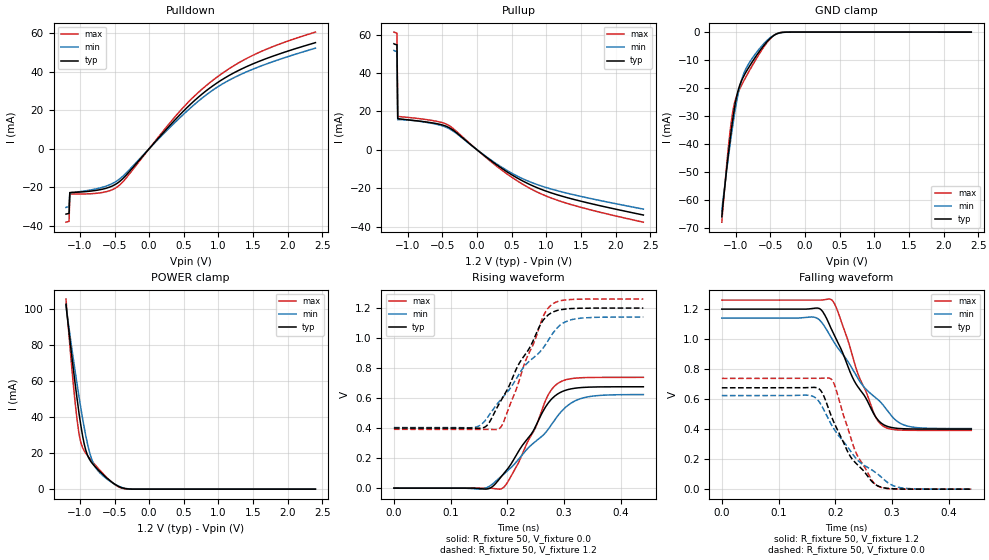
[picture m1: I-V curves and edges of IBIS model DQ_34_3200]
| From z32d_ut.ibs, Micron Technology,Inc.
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| MODEL DQ_34_3200 (34 Ohm Data I/O with no ODT, 1600-3200Mbps)
[Model]   DQ_34_3200
Model_type   I/O
Vinl = 905.000mV
Vinh = 1015.000mV
Vmeas = 960.000mV
Vref = 1200.000mV
Cref = 0.0pF
Rref = 50.000Ohm
|   typ   min   max
|C_comp   0.636pF   0.586pF   0.686pF
C_comp_pullup   0.318pF   0.293pF   0.343pF
C_comp_pulldown   0.318pF   0.293pF   0.343pF
[Model Spec]
| Timing spec test load voltage corners
Vref   1.2000V   1.1400V   1.2600V
| Dynamic Overshoot Parameters from DDR4 Specification
|D_overshoot_ampl_h   0.40   NA   NA
|D_overshoot_ampl_l   0.40   NA   NA
|D_overshoot_area_h   0.0800n   NA   NA
|D_overshoot_area_l   0.0800n   NA   NA
[Voltage Range]   1.2000V   1.1400V   1.2600V
| Junction Temperature (Ambient temp is 35C typ, 125C min, -40C max)
[Temperature Range]   50.0   140.0   -40.0
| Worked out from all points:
|   slope of the pulldown table from 0 to 0.18 V, typ, clamps not added: 24.5 ohm
|   slope of the pullup table from 0 to 0.18 V, typ, clamps not added: 35.6 ohm
|   GND clamp passes 1 mA (typ) near -0.44 V on its own axis
|   POWER clamp passes 1 mA (typ) near -0.41 V on its own axis
|   rising waveform, R_fixture 50, V_fixture 0.0: 20-80 % time 65.4ps typ, 89.5ps min, 51.3ps max; typ from 0 V to 0.675 V
|   rising waveform, R_fixture 50, V_fixture 1.2: 20-80 % time 66.8ps typ, 93.5ps min, 51.8ps max; typ from 0.4 V to 1.2 V
|   falling waveform, R_fixture 50, V_fixture 1.2: 20-80 % time 63.8ps typ, 90.8ps min, 48.9ps max; typ from 1.2 V to 0.4 V
|   falling waveform, R_fixture 50, V_fixture 0.0: 20-80 % time 59ps typ, 82.2ps min, 44.9ps max; typ from 0.676 V to 0 V
[Pulldown]
|   Voltage   I(typ)   I(min)   I(max)
-1.2V     -33.97mA   -30.5mA    -38.16mA
-1.156V   -33.6mA    -30.12mA   -37.79mA
-1.145V   -22.76mA   -22.9mA    -23.52mA
-676.4mV  -21.04mA   -20.05mA   -22.75mA
-545.5mV  -19.58mA   -18.32mA   -21.48mA
-436.4mV  -17.3mA    -15.97mA   -19.17mA
447.3mV   17.75mA    16.22mA    19.64mA
687.3mV   26.05mA    24.03mA    28.48mA
960mV     33.69mA    31.44mA    36.67mA
1.222V    39.38mA    36.85mA    43.11mA
1.527V    44.52mA    41.76mA    49.04mA
2.4V      55.1mA     52.23mA    60.58mA
[GND Clamp]
|   Voltage   I(typ)   I(min)   I(max)
-1.2V     -66.16mA   -64.28mA   -68.09mA
-1.135V   -50.09mA   -50.4mA    -48.84mA
-1.091V   -40.54mA   -42.05mA   -37.85mA
-1.047V   -32.06mA   -34.29mA   -29.28mA
-1.004V   -25.24mA   -27.37mA   -24.15mA
-960mV    -20.46mA   -21.61mA   -21.27mA
-916.4mV  -17.45mA   -17.25mA   -19.05mA
-840mV    -13.84mA   -12.54mA   -15.5mA
-643.6mV  -6.426mA   -5.55mA    -7.18mA
-458.2mV  -1.359mA   -1.253mA   -1.332mA
-250.9mV  -9.002uA   -25.19uA   1.741uA
2.4V      0A         0A         0A
[Pullup]
|   Voltage   I(typ)   I(min)   I(max)
-1.2V     55.21mA    51.74mA    61.29mA
-1.156V   54.64mA    51.12mA    60.76mA
-1.145V   16.26mA    15.68mA    17.4mA
-730.9mV  14.48mA    14.3mA     15.75mA
-523.6mV  13.17mA    12.73mA    14.37mA
-414.5mV  11.76mA    11.22mA    12.86mA
-316.4mV  9.458mA    9.031mA    10.21mA
370.9mV   -9.995mA   -9.387mA   -10.94mA
621.8mV   -15.5mA    -14.42mA   -17.08mA
949.1mV   -20.87mA   -19.07mA   -23.31mA
1.495V    -26.7mA    -24.21mA   -29.89mA
2.4V      -33.93mA   -30.84mA   -37.66mA
[POWER Clamp]
|   Voltage   I(typ)   I(min)   I(max)
-1.2V     102.5mA    102mA      105.3mA
-1.135V   79.77mA    83.1mA     75.19mA
-1.08V    62.13mA    68.42mA    52.54mA
-1.036V   48.91mA    57.17mA    37.32mA
-992.7mV  37.04mA    46.51mA    27.02mA
-916.4mV  21.89mA    29.93mA    20mA
-861.8mV  16.57mA    20.7mA     17.26mA
-807.3mV  13.63mA    14.48mA    14.72mA
-709.1mV  9.665mA    8.958mA    10.4mA
-512.7mV  3.198mA    3.102mA    3.061mA
-250.9mV  21.9uA     63.81uA    -1.736uA
2.4V      0A         0A         0A
[Ramp]
|   typ   min   max
| 20% - 80%
dV/dt_r   405.29m/65.42p   374.07m/89.53p   442.96m/51.27p
dV/dt_f   479.80m/63.86p   441.74m/90.76p   520.92m/48.87p
| Slew rate: Power terminated
|SR_r[V/ns]   7.18   4.73   10.05
|SR_f[V/ns]   7.51   4.87   10.66
| 25% - 75%
|dV/dt_r   337.74m/54.25p   311.72m/74.53p   369.13m/42.54p
|dV/dt_f   399.83m/53.48p   368.12m/76.15p   434.10m/40.83p
| Slew rate: Power terminated
|SR_r[V/ns]   7.13   4.64   9.99
|SR_f[V/ns]   7.48   4.83   10.63
R_load = 50
[Rising Waveform]
R_fixture = 50
V_fixture = 0.0
|   Time   V(typ)   V(min)   V(max)
0s        5.466uV    31.66uV    320nV
164ps     -6.16mV    3.513mV    348.8uV
190ps     79.57mV    81.73mV    -3.675mV
217ps     227.7mV    179.2mV    148mV
250ps     412.1mV    311.5mV    405.2mV
270ps     555.5mV    381.5mV    605.2mV
287ps     622.8mV    472mV      691.8mV
308ps     657.8mV    554.8mV    726.5mV
333ps     670.9mV    600.3mV    736.1mV
440ps     675.5mV    623.5mV    738.3mV
[Rising Waveform]
R_fixture   = 50
V_fixture   = 1.2
V_fixture_min = 1.14
V_fixture_max = 1.26
|   Time   V(typ)   V(min)   V(max)
0s        400.3mV    403.7mV    391.8mV
156ps     401mV      430.1mV    391.9mV
167ps     430.5mV    481.7mV    391.4mV
185ps     557.9mV    574.4mV    395.1mV
194ps     615.4mV    613.2mV    446mV
230ps     882.2mV    811.1mV    826.3mV
259ps     1.094V     914.1mV    1.102V
276ps     1.164V     1.008V     1.216V
316ps     1.197V     1.125V     1.258V
440ps     1.2V       1.14V      1.26V
[Falling Waveform]
R_fixture   = 50
V_fixture   = 1.2
V_fixture_min = 1.14
V_fixture_max = 1.26
|   Time   V(typ)   V(min)   V(max)
0s        1.2V       1.14V      1.26V
169ps     1.207V     1.137V     1.26V
192ps     1.077V     1.016V     1.265V
205ps     974.9mV    939.3mV    1.18V
233ps     725.6mV    783.4mV    853.4mV
268ps     502mV      620.4mV    507.4mV
281ps     440.7mV    576.2mV    430.7mV
306ps     406.8mV    462.2mV    396.1mV
326ps     401.9mV    422mV      392.5mV
440ps     400.3mV    403.7mV    391.8mV
[Falling Waveform]
R_fixture = 50
V_fixture = 0.0
|   Time   V(typ)   V(min)   V(max)
0s        675.5mV    623.6mV    738.3mV
167ps     676.4mV    603.1mV    738.1mV
178ps     635.8mV    543.1mV    739.9mV
191ps     507.9mV    444.8mV    738mV
200ps     426.2mV    388.4mV    682.6mV
224ps     235.1mV    270mV      385.9mV
236ps     175mV      207.8mV    248.3mV
272ps     28.24mV    109.3mV    28.54mV
315ps     904.6uV    10.04mV    411.5uV
440ps     5.568uV    37.22uV    4.257uV
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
